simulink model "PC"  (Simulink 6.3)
settings: Solver=ode23tb  StartTime=0.0  StopTime=3*3600  MaxStep=10  RelTol=1e-6  AbsTol=1e-6
InitFcn:
  | Exp_data;
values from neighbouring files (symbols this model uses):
  mG_in = 0.362    [Exp_data.m]    (also in slug_3DAE.m = u(2); slug_3D_lin.m = u(2); slug_3D_sim.m = u(2); s_slug.m)
  mL_in = 8.64    [Exp_data.m]    (also in slug_3DAE.m = u(3); slug_3D_lin.m = u(3); slug_3D_sim.m = u(3); s_slug.m)
libraries: simulink_extras x1

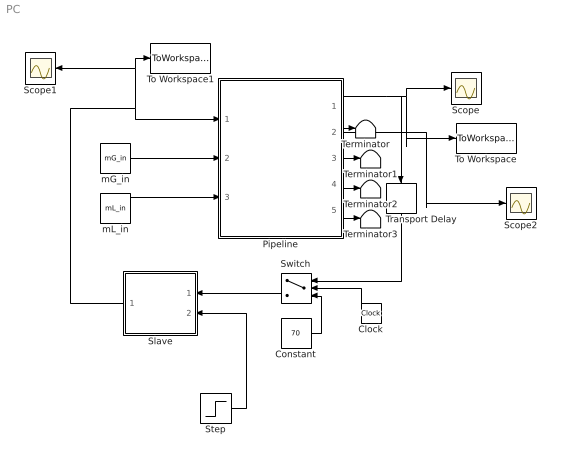
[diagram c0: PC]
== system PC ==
  Clock : Clock
  Constant : Constant  Value=70
  Pipeline : Subsystem
  Scope : Scope
  Scope1 : Scope
  Scope2 : Scope
  Slave : Subsystem  Orientation=left
  Step : Step  Time=3600  Before=70  After=70  SampleTime=0
  Switch : Switch  Orientation=left  Threshold=3600
  Terminator{,1..3} (4 alike) : Terminator
  To Workspace : ToWorkspace  VariableName=P1  SampleTime=-1  SaveFormat=Array
  To Workspace1 : ToWorkspace  VariableName=z  SampleTime=-1  SaveFormat=Array
  Transport Delay : TransportDelay  Orientation=down  InitialOutput=1
  mG_in : Constant  Value=mG_in
  mL_in : Constant  Value=mL_in
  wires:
  Pipeline/1(P1) -> Scope/1, To Workspace/1, Transport Delay/1
  Pipeline/2("P2 ") -> Terminator/1, Scope2/1
  Pipeline/3("rho_T ") -> Terminator1/1
  Pipeline/4(W) -> Terminator2/1
  Pipeline/5(Q) -> Terminator3/1
  mL_in/1 -> Pipeline/3(mL_in)
  mG_in/1 -> Pipeline/2(mG_in)
  Slave/1(z) -> Pipeline/1(z), To Workspace1/1, Scope1/1
  Clock/1 -> Switch/2
  Switch/1 -> Slave/1(measurement)
  Constant/1 -> Switch/3
  Transport Delay/1 -> Switch/1
  Step/1 -> Slave/2(ref)

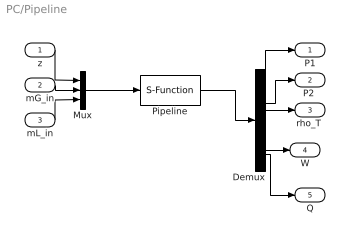
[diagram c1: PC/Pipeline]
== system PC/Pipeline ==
  z : Inport
  mG_in : Inport  Port=2
  mL_in : Inport  Port=3
  Demux : Demux  Outputs=5
  Mux : Mux  Inputs=3
  Pipeline : S-Function  FunctionName=s_slug
  P1 : Outport
  "P2 " : Outport  Port=2
  "rho_T " : Outport  Port=3
  W : Outport  Port=4
  Q : Outport  Port=5
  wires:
  Pipeline/1 -> Demux/1
  Mux/1 -> Pipeline/1
  Demux/1 -> P1/1
  z/1 -> Mux/1
  mG_in/1 -> Mux/2
  Demux/2 -> "P2 "/1
  mL_in/1 -> Mux/3
  Demux/3 -> "rho_T "/1
  Demux/4 -> W/1
  Demux/5 -> Q/1

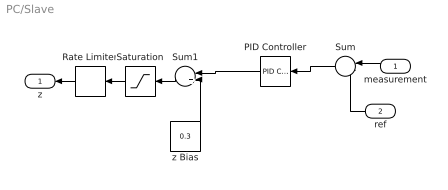
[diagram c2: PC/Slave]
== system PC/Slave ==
  measurement : Inport  Orientation=left
  ref : Inport  Orientation=left  Port=2
  PID Controller : simulink_extras/Additional Linear/PID Controller  Orientation=left  P=-0.5  I=-0.5/500  D=0
  Rate Limiter : RateLimiter  Orientation=left  RisingSlewLimit=1/60  FallingSlewLimit=-1/60
  Saturation : Saturate  Orientation=left  UpperLimit=1  LowerLimit=0.02
  Sum : Sum  Orientation=left  Inputs=|-+
  Sum1 : Sum  Orientation=left  Inputs=|++
  z Bias : Constant  Value=0.3
  z : Outport  Orientation=left
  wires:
  Sum/1 -> PID Controller/1
  z Bias/1 -> Sum1/2
  Sum1/1 -> Saturation/1
  measurement/1 -> Sum/1
  Saturation/1 -> Rate Limiter/1
  ref/1 -> Sum/2
  Rate Limiter/1 -> z/1
  PID Controller/1 -> Sum1/1
